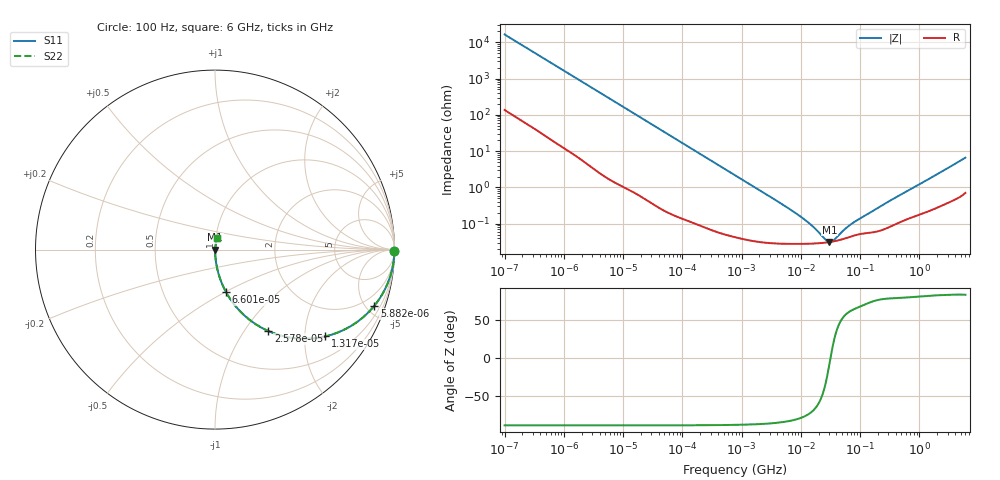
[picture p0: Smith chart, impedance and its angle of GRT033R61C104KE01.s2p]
!Murata Part Number: GRT033R61C104KE01
!These Parameters are Measured in Series Mode Connection
!Data Generated on Jun 19, 2026
!  o--ll--o
!Port1  Port2
!  o------o
!Operation Temp=25[degC], DC Bias Voltage=0[V]
!Freq. Start=100[Hz] Stop=6[GHz] 401[Steps]
# Hz S RI R 50
!Freq.(Hz) S11(Real) S11(Imag) S21(Real) S21(Imag) S12(Real) S12(Imag) S22(Real) S22(Imag)
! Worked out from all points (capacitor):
!   401 points, 100 Hz to 6 GHz, reference 50 ohm
!   read as one part in series: C = 97.3 nF near 109 Hz
!   lowest |Z| = 31.6 mohm at 30.45 MHz (marker M1)
!   series resonance near 31.72 MHz, so ESL is about 260 pH
!   S11 on the Smith chart (normalised r, x): 100 Hz: open; 5.882 kHz: 1.03, -5.65; 13.17 kHz: 1.02, -2.53; 25.78 kHz: 1.01, -1.30; 66 kHz: 1.00, -0.51; 6 GHz: 1.01, +0.13
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100  0.9999 -0.00613  8.87e-05 0.00613  8.87e-05 0.00613  0.9999 -0.00613
627  0.9983 -0.038  0.00173 0.038  0.00173 0.038  0.9983 -0.038
2008  0.9847 -0.1193  0.0153 0.1193  0.0153 0.1193  0.9847 -0.1193
3759  0.9501 -0.2148  0.0499 0.2148  0.0499 0.2148  0.9501 -0.2148
5882  0.8874 -0.3133  0.1126 0.3133  0.1126 0.3133  0.8874 -0.3133
8801  0.7802 -0.4111  0.2198 0.4111  0.2198 0.4111  0.7802 -0.4111
13169  0.6152 -0.4833  0.3848 0.4833  0.3848 0.4833  0.6152 -0.4833
18016  0.4624 -0.4952  0.5376 0.4952  0.5376 0.4952  0.4624 -0.4952
25777  0.2975 -0.4538  0.7025 0.4538  0.7025 0.4538  0.2975 -0.4538
40335  0.1488 -0.3526  0.8512 0.3526  0.8512 0.3526  0.1488 -0.3526
66005  0.0622 -0.238  0.9378 0.238  0.9378 0.238  0.0622 -0.238
184852  0.00915 -0.0902  0.9908 0.0902  0.9908 0.0902  0.00915 -0.0902
774597  0.000906 -0.0219  0.9991 0.0219  0.9991 0.0219  0.000906 -0.0219
6353432  0.000286 -0.00258  0.9997 0.00258  0.9997 0.00258  0.000286 -0.00258
1.555665e7  0.000285 -0.00083  0.9997 0.00083  0.9997 0.00083  0.000285 -0.00083
2.545746e7  0.000302 -0.000236  0.9997 0.000236  0.9997 0.000236  0.000302 -0.000236
3.045065e7  0.000313 -4.32e-05  0.9997 4.32e-05  0.9997 4.32e-05  0.000313 -4.32e-05
3.64232e7  0.00033 0.000145  0.9997 -0.000145  0.9997 -0.000145  0.00033 0.000145
5.449875e7  0.00039 0.000576  0.9996 -0.000576  0.9996 -0.000576  0.00039 0.000576
7.455971e7  0.00046 0.000931  0.9995 -0.000931  0.9995 -0.000931  0.00046 0.000931
3.124326e8  0.000828 0.00414  0.9992 -0.00414  0.9992 -0.00414  0.000828 0.00414
6e9  0.0113 0.0647  0.9887 -0.0647  0.9887 -0.0647  0.0113 0.0647
